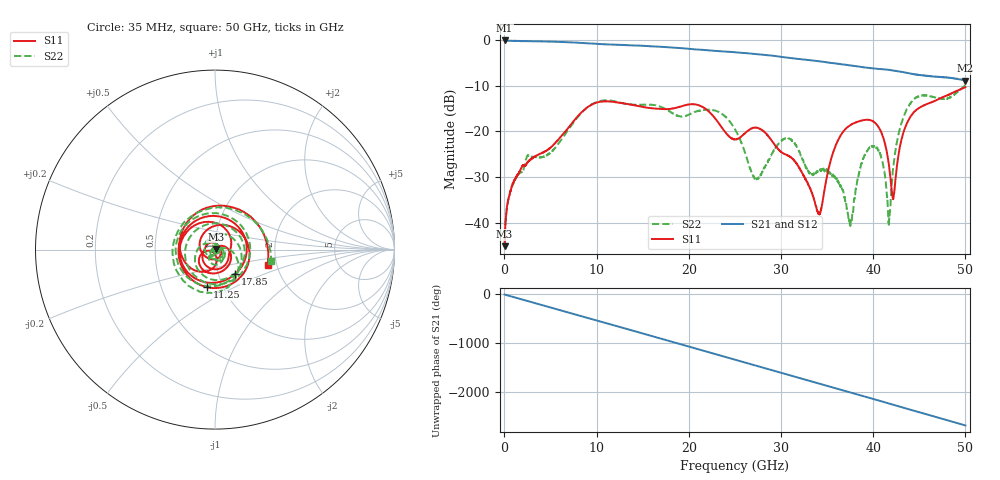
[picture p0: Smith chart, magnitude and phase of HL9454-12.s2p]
! 3/7/2022 11:38:54 AM
! H:\PRODUCTION_DATA\TEMP_S2P.S2P
! CHANNEL.1
! TR.MEASUREMENT
! CORRECTED.DATA
# GHZ S RI R 50.0
! FREQ.GHZ  S11RE  S11IM  S21RE  S21IM  S12RE  S12IM  S22RE  S22IM
!; PortSelection: Port_12
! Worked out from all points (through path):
!   3571 points, 35 MHz to 50 GHz, reference 50 ohm
!   highest |S21| = -0.04 dB at 35 MHz (marker M1); lowest = -8.8 dB at 49.97 GHz (marker M2)
!   group delay of S21, straight-line fit = 149 ps
!   lowest |S11| = -45.2 dB at 35 MHz (marker M3), VSWR 1.01, Z = 50.5 + j0.291 ohm
!   |S11| at or under -10 dB: start of sweep to end of sweep
!   |S22| runs from -45.1 to -9.9 dB; largest |S21 - S12| = 0.011
!   S11 on the Smith chart (normalised r, x): 35 MHz: 1.01, +0.01; 11.25 GHz: 0.84, -0.37; 17.85 GHz: 1.20, -0.34; 50 GHz: 1.79, -0.34
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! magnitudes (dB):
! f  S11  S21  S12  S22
! 35 MHz  -45.2  0.0  0.0  -45.1
! 776.8 MHz  -32.3  -0.1  -0.1  -32.2
! 2.484 GHz  -26.8  -0.2  -0.2  -25.4
! 8.376 GHz  -15.8  -0.6  -0.6  -15.9
! 11.25 GHz  -13.4  -0.9  -0.9  -13.2
! 16.7 GHz  -15.0  -1.4  -1.4  -14.4
! 17.85 GHz  -15.1  -1.5  -1.5  -15.5
! 21.31 GHz  -14.4  -2.1  -2.1  -15.4
! 25.03 GHz  -21.7  -2.6  -2.6  -19.6
! 27.21 GHz  -19.2  -3.0  -3.0  -30.1
! 30.63 GHz  -25.2  -3.8  -3.8  -21.4
! 33.36 GHz  -33.4  -4.4  -4.4  -29.4
! 34.23 GHz  -37.9  -4.6  -4.6  -28.4
! 35.74 GHz  -24.1  -5.0  -5.0  -29.7
! 37.5 GHz  -18.6  -5.5  -5.5  -40.5
! 38.86 GHz  -17.6  -5.9  -5.9  -26.3
! 40.23 GHz  -18.1  -6.2  -6.2  -23.3
! 41.69 GHz  -27.0  -6.5  -6.5  -39.8
! 42.2 GHz  -34.5  -6.6  -6.6  -27.5
! 43.8 GHz  -17.6  -7.2  -7.2  -14.5
! 49.97 GHz  -10.3  -8.8  -8.7  -10.0
! 50 GHz  -10.3  -8.8  -8.8  -9.9
